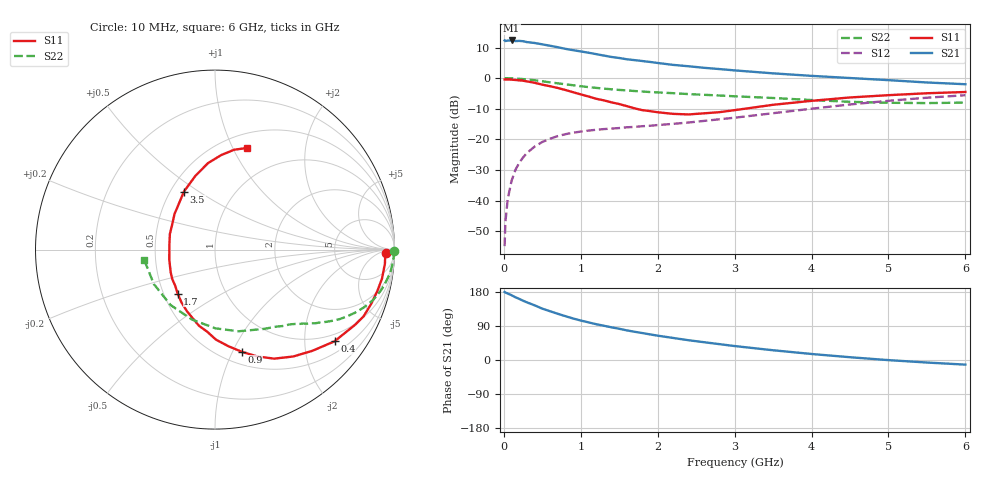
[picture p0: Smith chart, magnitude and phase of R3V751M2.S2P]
! SIEMENS Small Signal Semiconductors
! BFR181
! Si NPN RF Bipolar Junction Transistor in SOT23
! VCE = 0.75 V  IC = 1.2 mA
! Common Emitter S-Parameters:  May  1996
# GHz  S  MA  R  50
!  f  S11  S21  S12  S22
! GHz  MAG  ANG  MAG  ANG  MAG  ANG  MAG  ANG
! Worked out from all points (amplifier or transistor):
!   36 points, 10 MHz to 6 GHz, reference 50 ohm
!   highest |S21| = 12.3 dB at 100 MHz (marker M1)
!   |S21| within 3 dB of that: start of sweep to 860.9 MHz
!   unconditionally stable (mu >= 1): 1.777 GHz to 3.978 GHz
!   at 250 MHz: K = 0.18, MSG = 19.0 dB, |S12| = -25.9 dB
!   at 1.4 GHz: K = 0.86, MSG = 11.7 dB, |S12| = -16.5 dB
!   at 6 GHz: K = 0.93, MSG = 1.8 dB, |S12| = -5.6 dB
!   S11 on the Smith chart (normalised r, x): 10 MHz: 36, -13; 400 MHz: 0.79, -2.74; 900 MHz: 0.62, -1.09; 1.7 GHz: 0.59, -0.32; 3.5 GHz: 0.58, +0.44; 6 GHz: 0.65, +1.14
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0.01  0.9521 -1.0  4.122 179.4  0.0018 91.0  0.9967 -0.5
0.02  0.9491 -1.7  4.029 178.0  0.0044 87.5  0.9962 -1.0
0.05  0.9499 -4.8  4.105 175.5  0.0105 85.9  0.9966 -2.4
0.1  0.9444 -9.8  4.125 171.0  0.021 84.5  0.9918 -4.8
0.15  0.9334 -14.4  4.033 165.6  0.0316 79.9  0.985 -7.3
0.2  0.9208 -19.3  4.055 161.2  0.0414 77.7  0.9753 -9.4
0.25  0.9075 -24.2  4.01 156.5  0.0506 74.3  0.9645 -11.7
0.3  0.8848 -28.4  3.878 152.1  0.0599 72.3  0.9517 -13.9
0.4  0.8394 -37.5  3.753 144.3  0.0761 66.7  0.9236 -17.8
0.5  0.7826 -46.1  3.564 135.5  0.0906 62.3  0.8892 -21.3
0.6  0.738 -53.8  3.379 128.7  0.1023 58.2  0.8539 -24.4
0.7  0.6914 -61.5  3.2 122.0  0.113 54.6  0.8228 -27.0
0.9  0.5887 -75.3  2.864 109.5  0.1285 49.1  0.7656 -31.2
1.1  0.5016 -89.4  2.602 99.3  0.139 45.7  0.714 -34.6
1.4  0.4021 -108.0  2.217 86.2  0.15 42.4  0.6576 -38.9
1.7  0.3212 -130.4  1.968 74.5  0.1596 41.8  0.6156 -42.2
2.2  0.261 -167.4  1.646 58.2  0.1791 43.2  0.5679 -48.6
2.8  0.2778 148.8  1.408 41.9  0.2127 45.8  0.5206 -58.0
3.5  0.3668 118.1  1.197 25.7  0.2674 45.7  0.4737 -73.9
4.5  0.4835 94.6  1.004 7.3  0.3714 39.5  0.4102 -108.3
5.5  0.5662 79.2  0.849 -6.7  0.4788 27.5  0.3912 -150.6
6  0.5938 72.5  0.795 -12.2  0.5261 20.1  0.3983 -171.6
